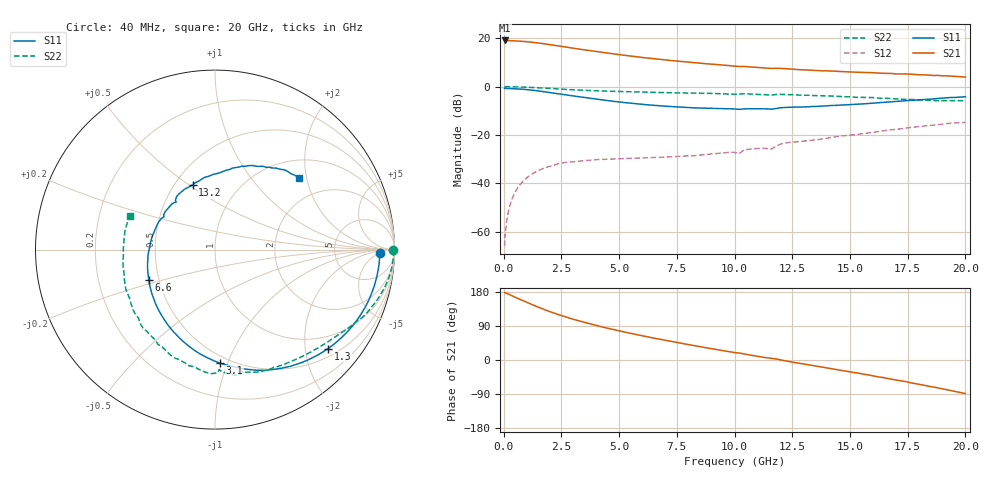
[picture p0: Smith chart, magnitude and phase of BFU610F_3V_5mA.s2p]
! Filename:  P:\Prog\Test\Noise\ATS_data\Testdata_Net\SplitFiles\BFU610_2W_A5_HighFreq_3V_5mA_D.s2p
! Date/Time: Wed 10/Aug/2011 16:57:20
! BFU610_2W_A5_HighFreq_3V_1mA_10mA_Bias3_R.s2p
! MDIF S-parameter v. bias file
! BFU610_2W_A5_HighFreq_3V_1mA_10mA
! Date/time Mon Aug 08 14:07:26 2011
! VAR V_out= 3.0000
! VAR I_out= 5.0000
! VAR V_in= 0.8932
! VAR I_in= 0.0399
! Device data file deembeded for feedlines and parallel
! Original file: \SplitFiles\BFU610_2W_A5_HighFreq_3V_5mA_R.s2p
! Feed-files: PR003V01_101208_Feed1.s2p, PR003V01_101208_Feed2.s2p
! Parallel-file: PR003V01_101208_Par.s2p
# MHz S MA R 50
!  Freq-MHz  S11-mag  S11-arg  S21-mag  S21-arg  S12-mag  S12-arg  S22-mag  S22-arg
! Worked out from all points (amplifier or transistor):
!   167 points, 40 MHz to 20 GHz, reference 50 ohm
!   highest |S21| = 19.1 dB at 40 MHz (marker M1)
!   |S21| within 3 dB of that: start of sweep to 2.886 GHz
!   unconditionally stable (mu >= 1): 5.137 GHz to 16.65 GHz
!   at 550 MHz: K = 0.05, MSG = 30.8 dB, |S12| = -42.7 dB
!   at 4.2 GHz: K = 0.80, MSG = 22.2 dB, |S12| = -30.1 dB
!   at 20 GHz: K = 0.78, MSG = 9.4 dB, |S12| = -14.8 dB
!   S11 on the Smith chart (normalised r, x): 40 MHz: 22, -6; 1.3 GHz: 0.68, -2.50; 3.1 GHz: 0.45, -0.94; 6.6 GHz: 0.44, -0.18; 13.2 GHz: 0.61, +0.52; 20 GHz: 1.40, +1.81
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40  0.9183 -1.2  8.985 178.2  0.0005037 86.3  0.9926 -0.2
60  0.9202 -1.7  8.963 177.5  0.000873 98.1  0.9941 -0.5
160  0.9176 -5.2  8.9 175.3  0.002034 89.2  0.9944 -1.9
400  0.9099 -13.1  8.879 168.5  0.005294 85.0  0.9915 -4.9
900  0.876 -29.1  8.549 154.6  0.01182 74.6  0.9745 -10.9
1300  0.8373 -41.2  8.175 144.2  0.01639 67.1  0.955 -15.4
1700  0.7928 -52.6  7.739 134.5  0.0202 60.5  0.9334 -19.5
2100  0.7453 -63.4  7.264 125.4  0.02325 54.9  0.9118 -23.3
2500  0.6967 -73.7  6.788 117.1  0.02615 49.7  0.8856 -26.8
3100  0.6325 -87.5  6.122 106.0  0.0282 43.1  0.8564 -31.4
3400  0.6036 -94.2  5.835 101.0  0.02923 41.1  0.8427 -33.5
4100  0.5429 -108.8  5.231 89.8  0.03107 37.0  0.8172 -38.1
4900  0.4871 -124.3  4.642 78.3  0.03225 34.3  0.7944 -43.4
5800  0.4387 -141.0  4.111 66.4  0.03333 33.0  0.7736 -49.3
6600  0.4063 -155.2  3.726 56.7  0.03439 32.9  0.7571 -54.4
6800  0.3998 -158.6  3.635 54.3  0.03463 33.2  0.7546 -55.7
8600  0.3595 171.7  3.027 34.2  0.03877 37.4  0.7291 -67.6
10200  0.3376 147.3  2.602 18.4  0.04133 42.1  0.6982 -77.0
13200  0.3824 109.0  2.198 -12.6  0.07601 37.5  0.6633 -102.6
13400  0.3883 106.9  2.166 -14.6  0.07842 36.7  0.6531 -104.8
16800  0.4881 72.1  1.87 -50.6  0.128 18.0  0.5657 -144.1
20000  0.6162 40.5  1.573 -88.5  0.1818 -13.4  0.5104 158.3
